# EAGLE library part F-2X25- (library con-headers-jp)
FEMALE HEADER
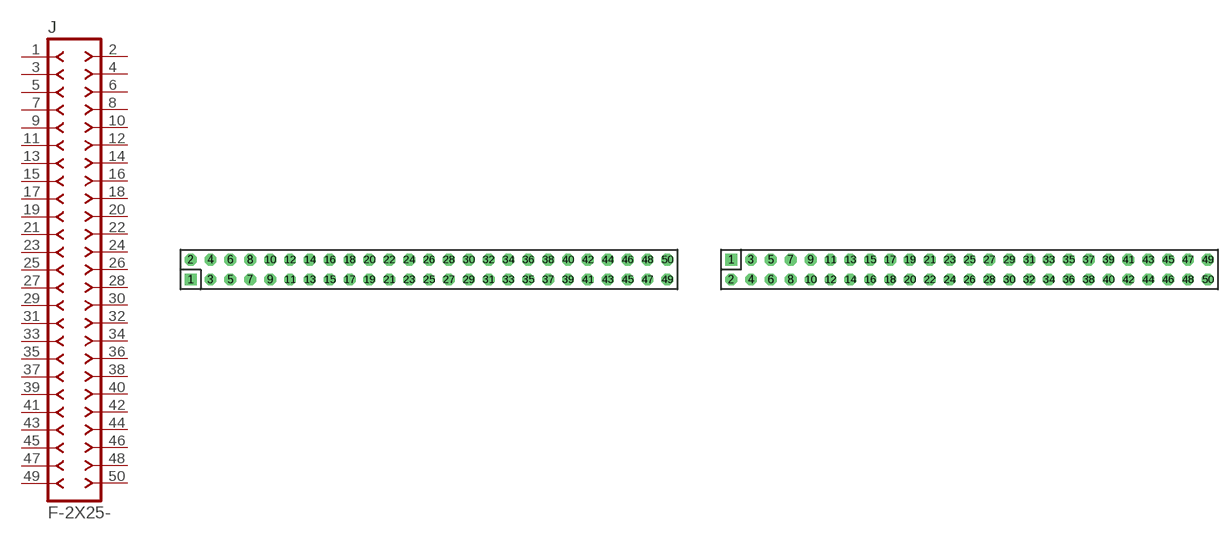
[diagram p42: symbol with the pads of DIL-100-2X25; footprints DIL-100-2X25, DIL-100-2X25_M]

Designator prefix J

## F-2X25-DIL-100  [DIL-100-2X25]
1  1  pas
2  2  pas
3  3  pas
4  4  pas
5  5  pas
6  6  pas
7  7  pas
8  8  pas
9  9  pas
10  10  pas
11  11  pas
12  12  pas
13  13  pas
14  14  pas
15  15  pas
16  16  pas
17  17  pas
18  18  pas
19  19  pas
20  20  pas
21  21  pas
22  22  pas
23  23  pas
24  24  pas
25  25  pas
26  26  pas
27  27  pas
28  28  pas
29  29  pas
30  30  pas
31  31  pas
32  32  pas
33  33  pas
34  34  pas
35  35  pas
36  36  pas
37  37  pas
38  38  pas
39  39  pas
40  40  pas
41  41  pas
42  42  pas
43  43  pas
44  44  pas
45  45  pas
46  46  pas
47  47  pas
48  48  pas
49  49  pas
50  50  pas

## F-2X25-DIL-100_M  [DIL-100-2X25_M]
Pads as for DIL-100-2X25

## F-2X25-DIL-2MM  [DIL-2MM-2X25]
Pads as for DIL-100-2X25

## F-2X25-DIL-2MM_M  [DIL-2MM-2X25_M]
Pads as for DIL-100-2X25

## Footprint DIL-100-2X25 (pad centres in mm)
PIN HEADER - 0.1"
drill 1.016 square: 1 -30.48,-1.27
drill 1.016 octagon: 2 -30.48,1.27; 3 -27.94,-1.27; 4 -27.94,1.27; 5 -25.4,-1.27; 6 -25.4,1.27; 7 -22.86,-1.27; 8 -22.86,1.27; 9 -20.32,-1.27; 10 -20.32,1.27; 11 -17.78,-1.27; 12 -17.78,1.27; 13 -15.24,-1.27; 14 -15.24,1.27; 15 -12.7,-1.27; 16 -12.7,1.27; 17 -10.16,-1.27; 18 -10.16,1.27; 19 -7.62,-1.27; 20 -7.62,1.27; 21 -5.08,-1.27; 22 -5.08,1.27; 23 -2.54,-1.27; 24 -2.54,1.27; 25 0,-1.27; 26 0,1.27; 27 2.54,-1.27; 28 2.54,1.27; 29 5.08,-1.27; 30 5.08,1.27; 31 7.62,-1.27; 32 7.62,1.27; 33 10.16,-1.27; 34 10.16,1.27; 35 12.7,-1.27; 36 12.7,1.27; 37 15.24,-1.27; 38 15.24,1.27; 39 17.78,-1.27; 40 17.78,1.27; 41 20.32,-1.27; 42 20.32,1.27; 43 22.86,-1.27; 44 22.86,1.27; 45 25.4,-1.27; 46 25.4,1.27; 47 27.94,-1.27; 48 27.94,1.27; 49 30.48,-1.27; 50 30.48,1.27

## Footprint DIL-100-2X25_M (pad centres in mm)
PIN HEADER - MIRRORED 0.1"
drill 1.016 square: 1 -30.48,1.27
drill 1.016 octagon: 2 -30.48,-1.27; 3 -27.94,1.27; 4 -27.94,-1.27; 5 -25.4,1.27; 6 -25.4,-1.27; 7 -22.86,1.27; 8 -22.86,-1.27; 9 -20.32,1.27; 10 -20.32,-1.27; 11 -17.78,1.27; 12 -17.78,-1.27; 13 -15.24,1.27; 14 -15.24,-1.27; 15 -12.7,1.27; 16 -12.7,-1.27; 17 -10.16,1.27; 18 -10.16,-1.27; 19 -7.62,1.27; 20 -7.62,-1.27; 21 -5.08,1.27; 22 -5.08,-1.27; 23 -2.54,1.27; 24 -2.54,-1.27; 25 0,1.27; 26 0,-1.27; 27 2.54,1.27; 28 2.54,-1.27; 29 5.08,1.27; 30 5.08,-1.27; 31 7.62,1.27; 32 7.62,-1.27; 33 10.16,1.27; 34 10.16,-1.27; 35 12.7,1.27; 36 12.7,-1.27; 37 15.24,1.27; 38 15.24,-1.27; 39 17.78,1.27; 40 17.78,-1.27; 41 20.32,1.27; 42 20.32,-1.27; 43 22.86,1.27; 44 22.86,-1.27; 45 25.4,1.27; 46 25.4,-1.27; 47 27.94,1.27; 48 27.94,-1.27; 49 30.48,1.27; 50 30.48,-1.27

## Footprint DIL-2MM-2X25 (pad centres in mm)
PIN HEADER - 2MM
drill 0.711 square: 1 -24,-1
drill 0.711: 2 -24,1; 3 -22,-1; 4 -22,1; 5 -20,-1; 6 -20,1; 7 -18,-1; 8 -18,1; 9 -16,-1; 10 -16,1; 11 -14,-1; 12 -14,1; 13 -12,-1; 14 -12,1; 15 -10,-1; 16 -10,1; 17 -8,-1; 18 -8,1; 19 -6,-1; 20 -6,1; 21 -4,-1; 22 -4,1; 23 -2,-1; 24 -2,1; 25 0,-1; 26 0,1; 27 2,-1; 28 2,1; 29 4,-1; 30 4,1; 31 6,-1; 32 6,1; 33 8,1; 34 8,-1; 35 10,1; 36 10,-1; 37 12,1; 38 12,-1; 39 14,1; 40 14,-1; 41 16,-1; 42 16,1; 43 18,-1; 44 18,1; 45 20,1; 46 20,-1; 47 22,1; 48 22,-1; 49 24,-1; 50 24,1

## Footprint DIL-2MM-2X25_M (pad centres in mm)
PIN HEADER - MIRRORED 2MM
drill 0.711 square: 1 -24,1
drill 0.711: 2 -24,-1; 3 -22,1; 4 -22,-1; 5 -20,1; 6 -20,-1; 7 -18,1; 8 -18,-1; 9 -16,1; 10 -16,-1; 11 -14,1; 12 -14,-1; 13 -12,1; 14 -12,-1; 15 -10,1; 16 -10,-1; 17 -8,1; 18 -8,-1; 19 -6,1; 20 -6,-1; 21 -4,1; 22 -4,-1; 23 -2,1; 24 -2,-1; 25 0,1; 26 0,-1; 27 2,1; 28 2,-1; 29 4,1; 30 4,-1; 31 6,1; 32 6,-1; 33 8,-1; 34 8,1; 35 10,-1; 36 10,1; 37 12,-1; 38 12,1; 39 14,-1; 40 14,1; 41 16,1; 42 16,-1; 43 18,1; 44 18,-1; 45 20,-1; 46 20,1; 47 22,-1; 48 22,1; 49 24,1; 50 24,-1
